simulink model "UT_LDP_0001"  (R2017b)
settings: Solver=FixedStepDiscrete  StartTime=0.0  StopTime=1  FixedStep=0.01  RelTol=1e-3  EnableMultiTasking=on
undefined symbols (not defined in the file): sigbuilder_block
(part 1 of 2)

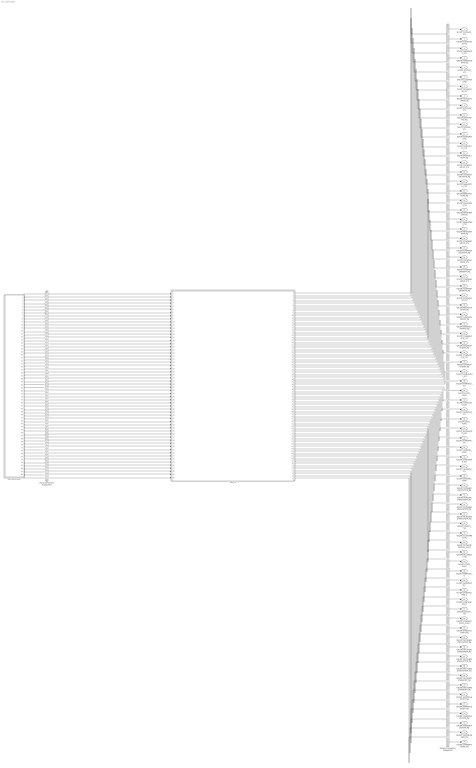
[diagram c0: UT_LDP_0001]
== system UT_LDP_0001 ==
  Harness Inputs : Subsystem  Tag=STV Subsys  LoadFcn=sigbuilder_block('load');  StartFcn=sigbuilder_block('start');  StopFcn=sigbuilder_block('stop');  ClipboardFcn=sigbuilder_block('clipboard');  mask(Sigbuilder block){tuvar=[0:10]}
      mask init:
      | if ~strcmp(get_param(bdroot(gcb),'SimulationStatus'),'stopped'),tuvar = sigbuilder_block('maskInit'); end
  Input Conversion Subsystem : Subsystem  Tag=__SLT_ICS__  Description=Signal spec. and routing
  LDP_UT : ModelReference  ModelNameDialog=LDP_UT  SimulationMode=Normal  ModelReferenceVersion='M104C110'
  Output Conversion Subsystem : Subsystem  Tag=__SLT_OCS__  Description=Signal spec. and routing
  GcLDP_CrntSens_mV : Outport  OutDataTypeStr=uint16  PortDimensions=[1]
  GbLDP_CrntSensVld_flg : Outport  Port=2  OutDataTypeStr=boolean  PortDimensions=[1]
  GcLDP_HallSplyVolt_mV : Outport  Port=3  OutDataTypeStr=uint16  PortDimensions=[1]
  GbLDP_HallSplyVoltVld_flg : Outport  Port=4  OutDataTypeStr=boolean  PortDimensions=[1]
  GcLDP_CC2Volt_mV : Outport  Port=5  OutDataTypeStr=uint16  PortDimensions=[1]
  GbLDP_CC2VoltVld_flg : Outport  Port=6  OutDataTypeStr=boolean  PortDimensions=[1]
  GcLDP_DCSuplyVolt_mV : Outport  Port=7  OutDataTypeStr=uint16  PortDimensions=[1]
  GbLDP_DCSuplyVoltVld_flg : Outport  Port=8  OutDataTypeStr=boolean  PortDimensions=[1]
  GcLDP_Kl30CVolt_mV : Outport  Port=9  OutDataTypeStr=uint16  PortDimensions=[1]
  GbLDP_Kl30CVoltVld_flg : Outport  Port=10  OutDataTypeStr=boolean  PortDimensions=[1]
  GcLDP_Kl30Volt_mV : Outport  Port=11  OutDataTypeStr=uint16  PortDimensions=[1]
  GbLDP_Kl30VoltVld_flg : Outport  Port=12  OutDataTypeStr=boolean  PortDimensions=[1]
  GcLDP_PosHsdCrnt_mV : Outport  Port=13  OutDataTypeStr=uint16  PortDimensions=[1]
  GbLDP_PosHsdCrntVld_flg : Outport  Port=14  OutDataTypeStr=boolean  PortDimensions=[1]
  GcLDP_ChrgPosHsdCrnt_mV : Outport  Port=15  OutDataTypeStr=uint16  PortDimensions=[1]
  GbLDP_ChrgPosHsdCrntVld_flg : Outport  Port=16  OutDataTypeStr=boolean  PortDimensions=[1]
  GcLDP_NegHsdCrnt_mV : Outport  Port=17  OutDataTypeStr=uint16  PortDimensions=[1]
  GbLDP_NegHsdCrntVld_flg : Outport  Port=18  OutDataTypeStr=boolean  PortDimensions=[1]
  GcLDP_PosHsdVolt_mV : Outport  Port=19  OutDataTypeStr=uint16  PortDimensions=[1]
  GbLDP_PosHsdVoltVld_flg : Outport  Port=20  OutDataTypeStr=boolean  PortDimensions=[1]
  GcLDP_NegHsdVolt_mV : Outport  Port=21  OutDataTypeStr=uint16  PortDimensions=[1]
  GbLDP_NegHsdVoltVld_flg : Outport  Port=22  OutDataTypeStr=boolean  PortDimensions=[1]
  GcLDP_ChrgNegHsdCrnt_mV : Outport  Port=23  OutDataTypeStr=uint16  PortDimensions=[1]
  GbLDP_ChrgNegHsdCrntVld_flg : Outport  Port=24  OutDataTypeStr=boolean  PortDimensions=[1]
  GcLDP_ChrgPosHsdVolt_mV : Outport  Port=25  OutDataTypeStr=uint16  PortDimensions=[1]
  GbLDP_ChrgPosHsdVoltVld_flg : Outport  Port=26  OutDataTypeStr=boolean  PortDimensions=[1]
  GcLDP_ChrgNegHsdVolt_mV : Outport  Port=27  OutDataTypeStr=uint16  PortDimensions=[1]
  GbLDP_ChrgNegHsdVoltVld_flg : Outport  Port=28  OutDataTypeStr=boolean  PortDimensions=[1]
  GcLDP_BmuSplyVolt_mV : Outport  Port=29  OutDataTypeStr=uint16  PortDimensions=[1]
  GbLDP_BmuSplyVoltVld_flg : Outport  Port=30  OutDataTypeStr=boolean  PortDimensions=[1]
  GbLDP_lntWtSensVoltVld_flg : Outport  Port=31  OutDataTypeStr=boolean  PortDimensions=[1]
  GbLDP_OutWtSensVoltVld_flg : Outport  Port=32  OutDataTypeStr=boolean  PortDimensions=[1]
  GcLDP_ChrgNegTemp_mV : Outport  Port=33  OutDataTypeStr=uint16  PortDimensions=[1]
  GbLDP_ChrgNegTempVld_flg : Outport  Port=34  OutDataTypeStr=boolean  PortDimensions=[1]
  GcLDP_ChrgPosTemp_mV : Outport  Port=35  OutDataTypeStr=uint16  PortDimensions=[1]
  GbLDP_ChrgPosTempVld_flg : Outport  Port=36  OutDataTypeStr=boolean  PortDimensions=[1]
  GcLDP_HvilDutyOut_pct : Outport  Port=37  OutDataTypeStr=uint8  PortDimensions=[1]
  GcLDP_HvilPerOut_ms : Outport  Port=38  OutDataTypeStr=uint32  PortDimensions=[1]
  GcLDP_HvilSt_numb : Outport  Port=39  OutDataTypeStr=uint8  PortDimensions=[1]
  GcLDP_CshDutyOut_pct : Outport  Port=40  OutDataTypeStr=uint8  PortDimensions=[1]
  GcLDP_CshPerOut_ms : Outport  Port=41  OutDataTypeStr=uint32  PortDimensions=[1]
  GcLDP_CshSt_numb : Outport  Port=42  OutDataTypeStr=uint8  PortDimensions=[1]
  GcLDP_HvilDutyFbkt_pct : Outport  Port=43  OutDataTypeStr=uint8  PortDimensions=[1]
  GcLDP_HvilPerFbk_ms : Outport  Port=44  OutDataTypeStr=uint32  PortDimensions=[1]
  GcLDP_HvilStFbk_numb : Outport  Port=45  OutDataTypeStr=uint8  PortDimensions=[1]
  GcLDP_CshDutyFbk_pct : Outport  Port=46  OutDataTypeStr=uint8  PortDimensions=[1]
  GcLDP_CshPerFbk_ms : Outport  Port=47  OutDataTypeStr=uint32  PortDimensions=[1]
  GcLDP_CshStFbk_numb : Outport  Port=48  OutDataTypeStr=uint8  PortDimensions=[1]
  GbLDP_DCPlugPosTempSTVFlt_flg : Outport  Port=49  OutDataTypeStr=boolean  PortDimensions=[1]
  GbLDP_DCPlugPosTempSTGFlt_flg : Outport  Port=50  OutDataTypeStr=boolean  PortDimensions=[1]
  GbLDP_DCPlugNegTempSTVFlt_flg : Outport  Port=51  OutDataTypeStr=boolean  PortDimensions=[1]
  GbLDP_DCPlugNegTempSTGFlt_flg : Outport  Port=52  OutDataTypeStr=boolean  PortDimensions=[1]
  GbLDP_CC2STG_flg : Outport  Port=53  OutDataTypeStr=boolean  PortDimensions=[1]
  GbLDP_CC2VoltRaty_flg : Outport  Port=54  OutDataTypeStr=boolean  PortDimensions=[1]
  GeLDP_DCPlugTempState_enum : Outport  Port=55  OutDataTypeStr=uint8  PortDimensions=[1]
  GbLDP_DC12VSply_flg : Outport  Port=56  OutDataTypeStr=boolean  PortDimensions=[1]
  GeLDP_CC2St_enum : Outport  Port=57  OutDataTypeStr=uint8  PortDimensions=[1]
  GcLDP_lntWtTemp_C : Outport  Port=58  OutDataTypeStr=single  PortDimensions=[1]
  GcLDP_OutWtTemp_C : Outport  Port=59  OutDataTypeStr=single  PortDimensions=[1]
  GcLDP_ChrgTempNeg_C : Outport  Port=60  OutDataTypeStr=single  PortDimensions=[1]
  GcLDP_ChrgTempPos_C : Outport  Port=61  OutDataTypeStr=single  PortDimensions=[1]
  GbLDP_CC2STV_flg : Outport  Port=62  OutDataTypeStr=boolean  PortDimensions=[1]
  GeLDP_ChrgGunConnSt_enum : Outport  Port=63  OutDataTypeStr=uint8  PortDimensions=[1]
  GbLDP_ChrgGunConnFlt_flg : Outport  Port=64  OutDataTypeStr=boolean  PortDimensions=[1]
  GbLDP_DCChrgPosTempSTVFlt_flg : Outport  Port=65  OutDataTypeStr=boolean  PortDimensions=[1]
  GbLDP_DCChrgPosTempSTGFlt_flg : Outport  Port=66  OutDataTypeStr=boolean  PortDimensions=[1]
  GbLDP_DCChrgNegTempSTVFlt_flg : Outport  Port=67  OutDataTypeStr=boolean  PortDimensions=[1]
  GbLDP_DCChrgNegTempSTGFlt_flg : Outport  Port=68  OutDataTypeStr=boolean  PortDimensions=[1]
  GbLDP_DCChrgPosTempHiFlt_flg : Outport  Port=69  OutDataTypeStr=boolean  PortDimensions=[1]
  GbLDP_DCChrgNegTempHiFlt_flg : Outport  Port=70  OutDataTypeStr=boolean  PortDimensions=[1]
  GbLDP_IntWtTempSTVFlt_flg : Outport  Port=71  OutDataTypeStr=boolean  PortDimensions=[1]
  GbLDP_IntWtTempSTGFlt_flg : Outport  Port=72  OutDataTypeStr=boolean  PortDimensions=[1]
  GbLDP_OutWtTempSTVFlt_flg : Outport  Port=73  OutDataTypeStr=boolean  PortDimensions=[1]
  GbLDP_OutWtTempSTGFlt_flg : Outport  Port=74  OutDataTypeStr=boolean  PortDimensions=[1]
  GbLDP_IntWtTempHiFlt_flg : Outport  Port=75  OutDataTypeStr=boolean  PortDimensions=[1]
  GbLDP_OutWtTempHiFlt_flg : Outport  Port=76  OutDataTypeStr=boolean  PortDimensions=[1]
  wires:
  Harness Inputs/1(GcISP_CrntSens_mV) -> Input Conversion Subsystem/1(Inport_1)
  Harness Inputs/2(GbISP_CrntSensL1Invld_flg) -> Input Conversion Subsystem/2(Inport_2)
  Harness Inputs/3(GbISP_HallSplyVoltVld_flg) -> Input Conversion Subsystem/3(Inport_3)
  Harness Inputs/4(GcISP_HallSplyVolt_mV) -> Input Conversion Subsystem/4(Inport_4)
  Harness Inputs/5(GcISP_CC2Volt_mV) -> Input Conversion Subsystem/5(Inport_5)
  Harness Inputs/6(GbISP_CC2VoltVld_flg) -> Input Conversion Subsystem/6(Inport_6)
  Harness Inputs/7(GcISP_DCSuplyVolt_mV) -> Input Conversion Subsystem/7(Inport_7)
  Harness Inputs/8(GbISP_DCSuplyVoltVld_flg) -> Input Conversion Subsystem/8(Inport_8)
  Harness Inputs/9(GcISP_Kl30CVolt_mV) -> Input Conversion Subsystem/9(Inport_9)
  Harness Inputs/10(GbISP_Kl30CVoltVld_flg) -> Input Conversion Subsystem/10(Inport_10)
  Harness Inputs/11(GbISP_Kl30VoltVld_flg) -> Input Conversion Subsystem/11(Inport_11)
  Harness Inputs/12(GcISP_Kl30Volt_mV) -> Input Conversion Subsystem/12(Inport_12)
  Harness Inputs/13(GcISP_PosHsdCrnt_mV) -> Input Conversion Subsystem/13(Inport_13)
  Harness Inputs/14(GbISP_PosHsdCrntVld_flg) -> Input Conversion Subsystem/14(Inport_14)
  Harness Inputs/15(GcISP_ChrgPosHsdCrnt_mV) -> Input Conversion Subsystem/15(Inport_15)
  Harness Inputs/16(GbISP_ChrgPosHsdCrntVld_flg) -> Input Conversion Subsystem/16(Inport_16)
  Harness Inputs/17(GcISP_NegHsdCrnt_mV) -> Input Conversion Subsystem/17(Inport_17)
  Harness Inputs/18(GbISP_NegHsdCrntVld_flg) -> Input Conversion Subsystem/18(Inport_18)
  Harness Inputs/19(GcISP_PosHsdVolt_mV) -> Input Conversion Subsystem/19(Inport_19)
  Harness Inputs/20(GbISP_PosHsdVoltVld_flg) -> Input Conversion Subsystem/20(Inport_20)
  Harness Inputs/21(GcISP_NegHsdVolt_mV) -> Input Conversion Subsystem/21(Inport_21)
  Harness Inputs/22(GbISP_NegHsdVoltVld_flg) -> Input Conversion Subsystem/22(Inport_22)
  Harness Inputs/23(GcISP_ChrgNegHsdCrnt_mV) -> Input Conversion Subsystem/23(Inport_23)
  Harness Inputs/24(GbISP_ChrgNegHsdCrntVld_flg) -> Input Conversion Subsystem/24(Inport_24)
  Harness Inputs/25(GcISP_ChrgPosHsdVolt_mV) -> Input Conversion Subsystem/25(Inport_25)
  Harness Inputs/26(GbISP_ChrgPosHsdVoltVld_flg) -> Input Conversion Subsystem/26(Inport_26)
  Harness Inputs/27(GcISP_ChrgNegHsdVolt_mV) -> Input Conversion Subsystem/27(Inport_27)
  Harness Inputs/28(GbISP_ChrgNegHsdVoltVld_flg) -> Input Conversion Subsystem/28(Inport_28)
  Harness Inputs/29(GcISP_BmuSplyVolt_mV) -> Input Conversion Subsystem/29(Inport_29)
  Harness Inputs/30(GbISP_BmuSplyVoltVld_flg) -> Input Conversion Subsystem/30(Inport_30)
  Harness Inputs/31(GcISP_lntWtSensVolt_mV) -> Input Conversion Subsystem/31(Inport_31)
  Harness Inputs/32(GbISP_lntWtSensVoltVld_flg) -> Input Conversion Subsystem/32(Inport_32)
  Harness Inputs/33(GcISP_OutWtSensVolt_mV) -> Input Conversion Subsystem/33(Inport_33)
  Harness Inputs/34(GbISP_OutWtSensVoltVld_flg) -> Input Conversion Subsystem/34(Inport_34)
  Harness Inputs/35(GcISP_ChrgNegTemp_mV) -> Input Conversion Subsystem/35(Inport_35)
  Harness Inputs/36(GbISP_ChrgNegTempVld_flg) -> Input Conversion Subsystem/36(Inport_36)
  Harness Inputs/37(GcISP_ChrgPosTemp_mV) -> Input Conversion Subsystem/37(Inport_37)
  Harness Inputs/38(GbISP_ChrgPosTempVld_flg) -> Input Conversion Subsystem/38(Inport_38)
  Harness Inputs/39(GcISP_HvilDutyOut_pct) -> Input Conversion Subsystem/39(Inport_39)
  Harness Inputs/40(GcISP_HvilPerOut_us) -> Input Conversion Subsystem/40(Inport_40)
  Harness Inputs/41(GcISP_HvilSt_numb) -> Input Conversion Subsystem/41(Inport_41)
  Harness Inputs/42(GbISP_HvilOutVld_flg) -> Input Conversion Subsystem/42(Inport_42)
  Harness Inputs/43(GcISP_CshDutyOut_pct) -> Input Conversion Subsystem/43(Inport_43)
  Harness Inputs/44(GcISP_CshPerOut_us) -> Input Conversion Subsystem/44(Inport_44)
  Harness Inputs/45(GcISP_CshSt_numb) -> Input Conversion Subsystem/45(Inport_45)
  Harness Inputs/46(GbISP_CshOutVld_flg) -> Input Conversion Subsystem/46(Inport_46)
  Harness Inputs/47(GcISP_HvilDutyFbkt_pct) -> Input Conversion Subsystem/47(Inport_47)
  Harness Inputs/48(GcISP_HvilPerFbk_us) -> Input Conversion Subsystem/48(Inport_48)
  Harness Inputs/49(GcISP_HvilStFbk_numb) -> Input Conversion Subsystem/49(Inport_49)
  Harness Inputs/50(GbISP_HvilFbkVld_flg) -> Input Conversion Subsystem/50(Inport_50)
  Harness Inputs/51(GcISP_CshDutyFbk_pct) -> Input Conversion Subsystem/51(Inport_51)
  Harness Inputs/52(GcISP_CshPerFbk_us) -> Input Conversion Subsystem/52(Inport_52)
  Harness Inputs/53(GcISP_CshStFbk_numb) -> Input Conversion Subsystem/53(Inport_53)
  Harness Inputs/54(GbISP_CshFbkVld_flg) -> Input Conversion Subsystem/54(Inport_54)
  Harness Inputs/55(GbISP_CrntSensL2Invld_flg) -> Input Conversion Subsystem/55(Inport_55)
  Harness Inputs/56(GeODP_ObcCcSt_enum) -> Input Conversion Subsystem/56(Inport_56)
  Harness Inputs/57(GbISP_TFCC2VoltRaty_flg) -> Input Conversion Subsystem/57(Inport_57)
  Harness Inputs/58(GbISP_TFCC2STV_flg) -> Input Conversion Subsystem/58(Inport_58)
  Harness Inputs/59(GbISP_TFCC2STG_flg) -> Input Conversion Subsystem/59(Inport_59)
  Harness Inputs/60(GeCTC_CtrCtlConnMode_enum) -> Input Conversion Subsystem/60(Inport_60)
  Output Conversion Subsystem/1(Outport_1) -> GcLDP_CrntSens_mV/1
  Output Conversion Subsystem/2(Outport_2) -> GbLDP_CrntSensVld_flg/1
  Output Conversion Subsystem/3(Outport_3) -> GcLDP_HallSplyVolt_mV/1
  Output Conversion Subsystem/4(Outport_4) -> GbLDP_HallSplyVoltVld_flg/1
  Output Conversion Subsystem/5(Outport_5) -> GcLDP_CC2Volt_mV/1
  Output Conversion Subsystem/6(Outport_6) -> GbLDP_CC2VoltVld_flg/1
  Output Conversion Subsystem/7(Outport_7) -> GcLDP_DCSuplyVolt_mV/1
  Output Conversion Subsystem/8(Outport_8) -> GbLDP_DCSuplyVoltVld_flg/1
  Output Conversion Subsystem/9(Outport_9) -> GcLDP_Kl30CVolt_mV/1
  Output Conversion Subsystem/10(Outport_10) -> GbLDP_Kl30CVoltVld_flg/1
  Output Conversion Subsystem/11(Outport_11) -> GcLDP_Kl30Volt_mV/1
  Output Conversion Subsystem/12(Outport_12) -> GbLDP_Kl30VoltVld_flg/1
  Output Conversion Subsystem/13(Outport_13) -> GcLDP_PosHsdCrnt_mV/1
  Output Conversion Subsystem/14(Outport_14) -> GbLDP_PosHsdCrntVld_flg/1
  Output Conversion Subsystem/15(Outport_15) -> GcLDP_ChrgPosHsdCrnt_mV/1
  Output Conversion Subsystem/16(Outport_16) -> GbLDP_ChrgPosHsdCrntVld_flg/1
  Output Conversion Subsystem/17(Outport_17) -> GcLDP_NegHsdCrnt_mV/1
  Output Conversion Subsystem/18(Outport_18) -> GbLDP_NegHsdCrntVld_flg/1
  Output Conversion Subsystem/19(Outport_19) -> GcLDP_PosHsdVolt_mV/1
  Output Conversion Subsystem/20(Outport_20) -> GbLDP_PosHsdVoltVld_flg/1
  Output Conversion Subsystem/21(Outport_21) -> GcLDP_NegHsdVolt_mV/1
  Output Conversion Subsystem/22(Outport_22) -> GbLDP_NegHsdVoltVld_flg/1
  Output Conversion Subsystem/23(Outport_23) -> GcLDP_ChrgNegHsdCrnt_mV/1
  Output Conversion Subsystem/24(Outport_24) -> GbLDP_ChrgNegHsdCrntVld_flg/1
  Output Conversion Subsystem/25(Outport_25) -> GcLDP_ChrgPosHsdVolt_mV/1
  Output Conversion Subsystem/26(Outport_26) -> GbLDP_ChrgPosHsdVoltVld_flg/1
  Output Conversion Subsystem/27(Outport_27) -> GcLDP_ChrgNegHsdVolt_mV/1
  Output Conversion Subsystem/28(Outport_28) -> GbLDP_ChrgNegHsdVoltVld_flg/1
  Output Conversion Subsystem/29(Outport_29) -> GcLDP_BmuSplyVolt_mV/1
  Output Conversion Subsystem/30(Outport_30) -> GbLDP_BmuSplyVoltVld_flg/1
  Output Conversion Subsystem/31(Outport_31) -> GbLDP_lntWtSensVoltVld_flg/1
  Output Conversion Subsystem/32(Outport_32) -> GbLDP_OutWtSensVoltVld_flg/1
  Output Conversion Subsystem/33(Outport_33) -> GcLDP_ChrgNegTemp_mV/1
  Output Conversion Subsystem/34(Outport_34) -> GbLDP_ChrgNegTempVld_flg/1
  Output Conversion Subsystem/35(Outport_35) -> GcLDP_ChrgPosTemp_mV/1
  Output Conversion Subsystem/36(Outport_36) -> GbLDP_ChrgPosTempVld_flg/1
  Output Conversion Subsystem/37(Outport_37) -> GcLDP_HvilDutyOut_pct/1
  Output Conversion Subsystem/38(Outport_38) -> GcLDP_HvilPerOut_ms/1
  Output Conversion Subsystem/39(Outport_39) -> GcLDP_HvilSt_numb/1
  Output Conversion Subsystem/40(Outport_40) -> GcLDP_CshDutyOut_pct/1
  Output Conversion Subsystem/41(Outport_41) -> GcLDP_CshPerOut_ms/1
  Output Conversion Subsystem/42(Outport_42) -> GcLDP_CshSt_numb/1
  Output Conversion Subsystem/43(Outport_43) -> GcLDP_HvilDutyFbkt_pct/1
  Output Conversion Subsystem/44(Outport_44) -> GcLDP_HvilPerFbk_ms/1
  Output Conversion Subsystem/45(Outport_45) -> GcLDP_HvilStFbk_numb/1
  Output Conversion Subsystem/46(Outport_46) -> GcLDP_CshDutyFbk_pct/1
  Output Conversion Subsystem/47(Outport_47) -> GcLDP_CshPerFbk_ms/1
  Output Conversion Subsystem/48(Outport_48) -> GcLDP_CshStFbk_numb/1
  Output Conversion Subsystem/49(Outport_49) -> GbLDP_DCPlugPosTempSTVFlt_flg/1
  Output Conversion Subsystem/50(Outport_50) -> GbLDP_DCPlugPosTempSTGFlt_flg/1
  Output Conversion Subsystem/51(Outport_51) -> GbLDP_DCPlugNegTempSTVFlt_flg/1
  Output Conversion Subsystem/52(Outport_52) -> GbLDP_DCPlugNegTempSTGFlt_flg/1
  Output Conversion Subsystem/53(Outport_53) -> GbLDP_CC2STG_flg/1
  Output Conversion Subsystem/54(Outport_54) -> GbLDP_CC2VoltRaty_flg/1
  Output Conversion Subsystem/55(Outport_55) -> GeLDP_DCPlugTempState_enum/1
  Output Conversion Subsystem/56(Outport_56) -> GbLDP_DC12VSply_flg/1
  Output Conversion Subsystem/57(Outport_57) -> GeLDP_CC2St_enum/1
  Output Conversion Subsystem/58(Outport_58) -> GcLDP_lntWtTemp_C/1
  Output Conversion Subsystem/59(Outport_59) -> GcLDP_OutWtTemp_C/1
  Output Conversion Subsystem/60(Outport_60) -> GcLDP_ChrgTempNeg_C/1
  Output Conversion Subsystem/61(Outport_61) -> GcLDP_ChrgTempPos_C/1
  Output Conversion Subsystem/62(Outport_62) -> GbLDP_CC2STV_flg/1
  Output Conversion Subsystem/63(Outport_63) -> GeLDP_ChrgGunConnSt_enum/1
  Output Conversion Subsystem/64(Outport_64) -> GbLDP_ChrgGunConnFlt_flg/1
  Output Conversion Subsystem/65(Outport_65) -> GbLDP_DCChrgPosTempSTVFlt_flg/1
  Output Conversion Subsystem/66(Outport_66) -> GbLDP_DCChrgPosTempSTGFlt_flg/1
  Output Conversion Subsystem/67(Outport_67) -> GbLDP_DCChrgNegTempSTVFlt_flg/1
  Output Conversion Subsystem/68(Outport_68) -> GbLDP_DCChrgNegTempSTGFlt_flg/1
  Output Conversion Subsystem/69(Outport_69) -> GbLDP_DCChrgPosTempHiFlt_flg/1
  Output Conversion Subsystem/70(Outport_70) -> GbLDP_DCChrgNegTempHiFlt_flg/1
  Output Conversion Subsystem/71(Outport_71) -> GbLDP_IntWtTempSTVFlt_flg/1
  Output Conversion Subsystem/72(Outport_72) -> GbLDP_IntWtTempSTGFlt_flg/1
  Output Conversion Subsystem/73(Outport_73) -> GbLDP_OutWtTempSTVFlt_flg/1
  Output Conversion Subsystem/74(Outport_74) -> GbLDP_OutWtTempSTGFlt_flg/1
  Output Conversion Subsystem/75(Outport_75) -> GbLDP_IntWtTempHiFlt_flg/1
  Output Conversion Subsystem/76(Outport_76) -> GbLDP_OutWtTempHiFlt_flg/1
  Input Conversion Subsystem/1(Outport_1) -> LDP_UT/1
  Input Conversion Subsystem/2(Outport_2) -> LDP_UT/2
  Input Conversion Subsystem/3(Outport_3) -> LDP_UT/3
  Input Conversion Subsystem/4(Outport_4) -> LDP_UT/4
  Input Conversion Subsystem/5(Outport_5) -> LDP_UT/5
  Input Conversion Subsystem/6(Outport_6) -> LDP_UT/6
  Input Conversion Subsystem/7(Outport_7) -> LDP_UT/7
  Input Conversion Subsystem/8(Outport_8) -> LDP_UT/8
  Input Conversion Subsystem/9(Outport_9) -> LDP_UT/9
  Input Conversion Subsystem/10(Outport_10) -> LDP_UT/10
  Input Conversion Subsystem/11(Outport_11) -> LDP_UT/11
  Input Conversion Subsystem/12(Outport_12) -> LDP_UT/12
  Input Conversion Subsystem/13(Outport_13) -> LDP_UT/13
  Input Conversion Subsystem/14(Outport_14) -> LDP_UT/14
  Input Conversion Subsystem/15(Outport_15) -> LDP_UT/15
  Input Conversion Subsystem/16(Outport_16) -> LDP_UT/16
  Input Conversion Subsystem/17(Outport_17) -> LDP_UT/17
  Input Conversion Subsystem/18(Outport_18) -> LDP_UT/18
  Input Conversion Subsystem/19(Outport_19) -> LDP_UT/19
  Input Conversion Subsystem/20(Outport_20) -> LDP_UT/20
  Input Conversion Subsystem/21(Outport_21) -> LDP_UT/21
  Input Conversion Subsystem/22(Outport_22) -> LDP_UT/22
  Input Conversion Subsystem/23(Outport_23) -> LDP_UT/23
  Input Conversion Subsystem/24(Outport_24) -> LDP_UT/24
  Input Conversion Subsystem/25(Outport_25) -> LDP_UT/25
  Input Conversion Subsystem/26(Outport_26) -> LDP_UT/26
  Input Conversion Subsystem/27(Outport_27) -> LDP_UT/27
  Input Conversion Subsystem/28(Outport_28) -> LDP_UT/28
  Input Conversion Subsystem/29(Outport_29) -> LDP_UT/29
  Input Conversion Subsystem/30(Outport_30) -> LDP_UT/30
  Input Conversion Subsystem/31(Outport_31) -> LDP_UT/31
  Input Conversion Subsystem/32(Outport_32) -> LDP_UT/32
  Input Conversion Subsystem/33(Outport_33) -> LDP_UT/33
  Input Conversion Subsystem/34(Outport_34) -> LDP_UT/34
  Input Conversion Subsystem/35(Outport_35) -> LDP_UT/35
  Input Conversion Subsystem/36(Outport_36) -> LDP_UT/36
  Input Conversion Subsystem/37(Outport_37) -> LDP_UT/37
  Input Conversion Subsystem/38(Outport_38) -> LDP_UT/38
  Input Conversion Subsystem/39(Outport_39) -> LDP_UT/39
  Input Conversion Subsystem/40(Outport_40) -> LDP_UT/40
  Input Conversion Subsystem/41(Outport_41) -> LDP_UT/41
  Input Conversion Subsystem/42(Outport_42) -> LDP_UT/42
  Input Conversion Subsystem/43(Outport_43) -> LDP_UT/43
  Input Conversion Subsystem/44(Outport_44) -> LDP_UT/44
  Input Conversion Subsystem/45(Outport_45) -> LDP_UT/45
  Input Conversion Subsystem/46(Outport_46) -> LDP_UT/46
  Input Conversion Subsystem/47(Outport_47) -> LDP_UT/47
  Input Conversion Subsystem/48(Outport_48) -> LDP_UT/48
  Input Conversion Subsystem/49(Outport_49) -> LDP_UT/49
  Input Conversion Subsystem/50(Outport_50) -> LDP_UT/50
  Input Conversion Subsystem/51(Outport_51) -> LDP_UT/51
  Input Conversion Subsystem/52(Outport_52) -> LDP_UT/52
  Input Conversion Subsystem/53(Outport_53) -> LDP_UT/53
  Input Conversion Subsystem/54(Outport_54) -> LDP_UT/54
  Input Conversion Subsystem/55(Outport_55) -> LDP_UT/55
  Input Conversion Subsystem/56(Outport_56) -> LDP_UT/56
  Input Conversion Subsystem/57(Outport_57) -> LDP_UT/57
  Input Conversion Subsystem/58(Outport_58) -> LDP_UT/58
  Input Conversion Subsystem/59(Outport_59) -> LDP_UT/59
  Input Conversion Subsystem/60(Outport_60) -> LDP_UT/60
  LDP_UT/1 -> Output Conversion Subsystem/1(Inport_1)
  LDP_UT/2 -> Output Conversion Subsystem/2(Inport_2)
  LDP_UT/3 -> Output Conversion Subsystem/3(Inport_3)
  LDP_UT/4 -> Output Conversion Subsystem/4(Inport_4)
  LDP_UT/5 -> Output Conversion Subsystem/5(Inport_5)
  LDP_UT/6 -> Output Conversion Subsystem/6(Inport_6)
  LDP_UT/7 -> Output Conversion Subsystem/7(Inport_7)
  LDP_UT/8 -> Output Conversion Subsystem/8(Inport_8)
  LDP_UT/9 -> Output Conversion Subsystem/9(Inport_9)
  LDP_UT/10 -> Output Conversion Subsystem/10(Inport_10)
  LDP_UT/11 -> Output Conversion Subsystem/11(Inport_11)
  LDP_UT/12 -> Output Conversion Subsystem/12(Inport_12)
  LDP_UT/13 -> Output Conversion Subsystem/13(Inport_13)
  LDP_UT/14 -> Output Conversion Subsystem/14(Inport_14)
  LDP_UT/15 -> Output Conversion Subsystem/15(Inport_15)
  LDP_UT/16 -> Output Conversion Subsystem/16(Inport_16)
  LDP_UT/17 -> Output Conversion Subsystem/17(Inport_17)
  LDP_UT/18 -> Output Conversion Subsystem/18(Inport_18)
  LDP_UT/19 -> Output Conversion Subsystem/19(Inport_19)
  LDP_UT/20 -> Output Conversion Subsystem/20(Inport_20)
  LDP_UT/21 -> Output Conversion Subsystem/21(Inport_21)
  LDP_UT/22 -> Output Conversion Subsystem/22(Inport_22)
  LDP_UT/23 -> Output Conversion Subsystem/23(Inport_23)
  LDP_UT/24 -> Output Conversion Subsystem/24(Inport_24)
  LDP_UT/25 -> Output Conversion Subsystem/25(Inport_25)
  LDP_UT/26 -> Output Conversion Subsystem/26(Inport_26)
  LDP_UT/27 -> Output Conversion Subsystem/27(Inport_27)
  LDP_UT/28 -> Output Conversion Subsystem/28(Inport_28)
  LDP_UT/29 -> Output Conversion Subsystem/29(Inport_29)
  LDP_UT/30 -> Output Conversion Subsystem/30(Inport_30)
  LDP_UT/31 -> Output Conversion Subsystem/31(Inport_31)
  LDP_UT/32 -> Output Conversion Subsystem/32(Inport_32)
  LDP_UT/33 -> Output Conversion Subsystem/33(Inport_33)
  LDP_UT/34 -> Output Conversion Subsystem/34(Inport_34)
  LDP_UT/35 -> Output Conversion Subsystem/35(Inport_35)
  LDP_UT/36 -> Output Conversion Subsystem/36(Inport_36)
  LDP_UT/37 -> Output Conversion Subsystem/37(Inport_37)
  LDP_UT/38 -> Output Conversion Subsystem/38(Inport_38)
  LDP_UT/39 -> Output Conversion Subsystem/39(Inport_39)
  LDP_UT/40 -> Output Conversion Subsystem/40(Inport_40)
  LDP_UT/41 -> Output Conversion Subsystem/41(Inport_41)
  LDP_UT/42 -> Output Conversion Subsystem/42(Inport_42)
  LDP_UT/43 -> Output Conversion Subsystem/43(Inport_43)
  LDP_UT/44 -> Output Conversion Subsystem/44(Inport_44)
  LDP_UT/45 -> Output Conversion Subsystem/45(Inport_45)
  LDP_UT/46 -> Output Conversion Subsystem/46(Inport_46)
  LDP_UT/47 -> Output Conversion Subsystem/47(Inport_47)
  LDP_UT/48 -> Output Conversion Subsystem/48(Inport_48)
  LDP_UT/49 -> Output Conversion Subsystem/49(Inport_49)
  LDP_UT/50 -> Output Conversion Subsystem/50(Inport_50)
  LDP_UT/51 -> Output Conversion Subsystem/51(Inport_51)
  LDP_UT/52 -> Output Conversion Subsystem/52(Inport_52)
  LDP_UT/53 -> Output Conversion Subsystem/53(Inport_53)
  LDP_UT/54 -> Output Conversion Subsystem/54(Inport_54)
  LDP_UT/55 -> Output Conversion Subsystem/55(Inport_55)
  LDP_UT/56 -> Output Conversion Subsystem/56(Inport_56)
  LDP_UT/57 -> Output Conversion Subsystem/57(Inport_57)
  LDP_UT/58 -> Output Conversion Subsystem/58(Inport_58)
  LDP_UT/59 -> Output Conversion Subsystem/59(Inport_59)
  LDP_UT/60 -> Output Conversion Subsystem/60(Inport_60)
  LDP_UT/61 -> Output Conversion Subsystem/61(Inport_61)
  LDP_UT/62 -> Output Conversion Subsystem/62(Inport_62)
  LDP_UT/63 -> Output Conversion Subsystem/63(Inport_63)
  LDP_UT/64 -> Output Conversion Subsystem/64(Inport_64)
  LDP_UT/65 -> Output Conversion Subsystem/65(Inport_65)
  LDP_UT/66 -> Output Conversion Subsystem/66(Inport_66)
  LDP_UT/67 -> Output Conversion Subsystem/67(Inport_67)
  LDP_UT/68 -> Output Conversion Subsystem/68(Inport_68)
  LDP_UT/69 -> Output Conversion Subsystem/69(Inport_69)
  LDP_UT/70 -> Output Conversion Subsystem/70(Inport_70)
  LDP_UT/71 -> Output Conversion Subsystem/71(Inport_71)
  LDP_UT/72 -> Output Conversion Subsystem/72(Inport_72)
  LDP_UT/73 -> Output Conversion Subsystem/73(Inport_73)
  LDP_UT/74 -> Output Conversion Subsystem/74(Inport_74)
  LDP_UT/75 -> Output Conversion Subsystem/75(Inport_75)
  LDP_UT/76 -> Output Conversion Subsystem/76(Inport_76)

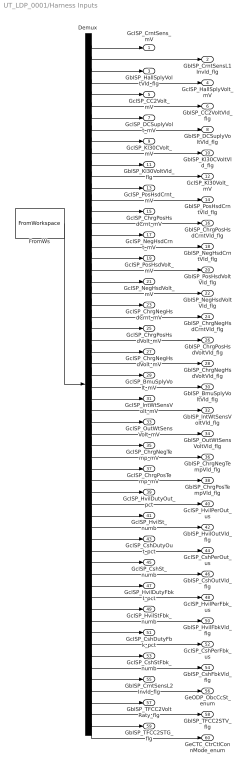
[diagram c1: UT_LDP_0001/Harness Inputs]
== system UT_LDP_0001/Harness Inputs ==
  Demux : Demux  Tag=STV Demux  Outputs=60
  FromWs : FromWorkspace  Tag=STV FromWs  VariableName=tuvar  SampleTime=0
  GcISP_CrntSens_mV : Outport  Tag=STV Outport
  GbISP_CrntSensL1Invld_flg : Outport  Tag=STV Outport  Port=2
  GbISP_HallSplyVoltVld_flg : Outport  Tag=STV Outport  Port=3
  GcISP_HallSplyVolt_mV : Outport  Tag=STV Outport  Port=4
  GcISP_CC2Volt_mV : Outport  Tag=STV Outport  Port=5
  GbISP_CC2VoltVld_flg : Outport  Tag=STV Outport  Port=6
  GcISP_DCSuplyVolt_mV : Outport  Tag=STV Outport  Port=7
  GbISP_DCSuplyVoltVld_flg : Outport  Tag=STV Outport  Port=8
  GcISP_Kl30CVolt_mV : Outport  Tag=STV Outport  Port=9
  GbISP_Kl30CVoltVld_flg : Outport  Tag=STV Outport  Port=10
  GbISP_Kl30VoltVld_flg : Outport  Tag=STV Outport  Port=11
  GcISP_Kl30Volt_mV : Outport  Tag=STV Outport  Port=12
  GcISP_PosHsdCrnt_mV : Outport  Tag=STV Outport  Port=13
  GbISP_PosHsdCrntVld_flg : Outport  Tag=STV Outport  Port=14
  GcISP_ChrgPosHsdCrnt_mV : Outport  Tag=STV Outport  Port=15
  GbISP_ChrgPosHsdCrntVld_flg : Outport  Tag=STV Outport  Port=16
  GcISP_NegHsdCrnt_mV : Outport  Tag=STV Outport  Port=17
  GbISP_NegHsdCrntVld_flg : Outport  Tag=STV Outport  Port=18
  GcISP_PosHsdVolt_mV : Outport  Tag=STV Outport  Port=19
  GbISP_PosHsdVoltVld_flg : Outport  Tag=STV Outport  Port=20
  GcISP_NegHsdVolt_mV : Outport  Tag=STV Outport  Port=21
  GbISP_NegHsdVoltVld_flg : Outport  Tag=STV Outport  Port=22
  GcISP_ChrgNegHsdCrnt_mV : Outport  Tag=STV Outport  Port=23
  GbISP_ChrgNegHsdCrntVld_flg : Outport  Tag=STV Outport  Port=24
  GcISP_ChrgPosHsdVolt_mV : Outport  Tag=STV Outport  Port=25
  GbISP_ChrgPosHsdVoltVld_flg : Outport  Tag=STV Outport  Port=26
  GcISP_ChrgNegHsdVolt_mV : Outport  Tag=STV Outport  Port=27
  GbISP_ChrgNegHsdVoltVld_flg : Outport  Tag=STV Outport  Port=28
  GcISP_BmuSplyVolt_mV : Outport  Tag=STV Outport  Port=29
  GbISP_BmuSplyVoltVld_flg : Outport  Tag=STV Outport  Port=30
  GcISP_lntWtSensVolt_mV : Outport  Tag=STV Outport  Port=31
  GbISP_lntWtSensVoltVld_flg : Outport  Tag=STV Outport  Port=32
  GcISP_OutWtSensVolt_mV : Outport  Tag=STV Outport  Port=33
  GbISP_OutWtSensVoltVld_flg : Outport  Tag=STV Outport  Port=34
  GcISP_ChrgNegTemp_mV : Outport  Tag=STV Outport  Port=35
  GbISP_ChrgNegTempVld_flg : Outport  Tag=STV Outport  Port=36
  GcISP_ChrgPosTemp_mV : Outport  Tag=STV Outport  Port=37
  GbISP_ChrgPosTempVld_flg : Outport  Tag=STV Outport  Port=38
  GcISP_HvilDutyOut_pct : Outport  Tag=STV Outport  Port=39
  GcISP_HvilPerOut_us : Outport  Tag=STV Outport  Port=40
  GcISP_HvilSt_numb : Outport  Tag=STV Outport  Port=41
  GbISP_HvilOutVld_flg : Outport  Tag=STV Outport  Port=42
  GcISP_CshDutyOut_pct : Outport  Tag=STV Outport  Port=43
  GcISP_CshPerOut_us : Outport  Tag=STV Outport  Port=44
  GcISP_CshSt_numb : Outport  Tag=STV Outport  Port=45
  GbISP_CshOutVld_flg : Outport  Tag=STV Outport  Port=46
  GcISP_HvilDutyFbkt_pct : Outport  Tag=STV Outport  Port=47
  GcISP_HvilPerFbk_us : Outport  Tag=STV Outport  Port=48
  GcISP_HvilStFbk_numb : Outport  Tag=STV Outport  Port=49
  GbISP_HvilFbkVld_flg : Outport  Tag=STV Outport  Port=50
  GcISP_CshDutyFbk_pct : Outport  Tag=STV Outport  Port=51
  GcISP_CshPerFbk_us : Outport  Tag=STV Outport  Port=52
  GcISP_CshStFbk_numb : Outport  Tag=STV Outport  Port=53
  GbISP_CshFbkVld_flg : Outport  Tag=STV Outport  Port=54
  GbISP_CrntSensL2Invld_flg : Outport  Tag=STV Outport  Port=55
  GeODP_ObcCcSt_enum : Outport  Tag=STV Outport  Port=56
  GbISP_TFCC2VoltRaty_flg : Outport  Tag=STV Outport  Port=57
  GbISP_TFCC2STV_flg : Outport  Tag=STV Outport  Port=58
  GbISP_TFCC2STG_flg : Outport  Tag=STV Outport  Port=59
  GeCTC_CtrCtlConnMode_enum : Outport  Tag=STV Outport  Port=60
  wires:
  FromWs/1 -> Demux/1
  Demux/1 -> GcISP_CrntSens_mV/1
  Demux/2 -> GbISP_CrntSensL1Invld_flg/1
  Demux/3 -> GbISP_HallSplyVoltVld_flg/1
  Demux/4 -> GcISP_HallSplyVolt_mV/1
  Demux/5 -> GcISP_CC2Volt_mV/1
  Demux/6 -> GbISP_CC2VoltVld_flg/1
  Demux/7 -> GcISP_DCSuplyVolt_mV/1
  Demux/8 -> GbISP_DCSuplyVoltVld_flg/1
  Demux/9 -> GcISP_Kl30CVolt_mV/1
  Demux/10 -> GbISP_Kl30CVoltVld_flg/1
  Demux/11 -> GbISP_Kl30VoltVld_flg/1
  Demux/12 -> GcISP_Kl30Volt_mV/1
  Demux/13 -> GcISP_PosHsdCrnt_mV/1
  Demux/14 -> GbISP_PosHsdCrntVld_flg/1
  Demux/15 -> GcISP_ChrgPosHsdCrnt_mV/1
  Demux/16 -> GbISP_ChrgPosHsdCrntVld_flg/1
  Demux/17 -> GcISP_NegHsdCrnt_mV/1
  Demux/18 -> GbISP_NegHsdCrntVld_flg/1
  Demux/19 -> GcISP_PosHsdVolt_mV/1
  Demux/20 -> GbISP_PosHsdVoltVld_flg/1
  Demux/21 -> GcISP_NegHsdVolt_mV/1
  Demux/22 -> GbISP_NegHsdVoltVld_flg/1
  Demux/23 -> GcISP_ChrgNegHsdCrnt_mV/1
  Demux/24 -> GbISP_ChrgNegHsdCrntVld_flg/1
  Demux/25 -> GcISP_ChrgPosHsdVolt_mV/1
  Demux/26 -> GbISP_ChrgPosHsdVoltVld_flg/1
  Demux/27 -> GcISP_ChrgNegHsdVolt_mV/1
  Demux/28 -> GbISP_ChrgNegHsdVoltVld_flg/1
  Demux/29 -> GcISP_BmuSplyVolt_mV/1
  Demux/30 -> GbISP_BmuSplyVoltVld_flg/1
  Demux/31 -> GcISP_lntWtSensVolt_mV/1
  Demux/32 -> GbISP_lntWtSensVoltVld_flg/1
  Demux/33 -> GcISP_OutWtSensVolt_mV/1
  Demux/34 -> GbISP_OutWtSensVoltVld_flg/1
  Demux/35 -> GcISP_ChrgNegTemp_mV/1
  Demux/36 -> GbISP_ChrgNegTempVld_flg/1
  Demux/37 -> GcISP_ChrgPosTemp_mV/1
  Demux/38 -> GbISP_ChrgPosTempVld_flg/1
  Demux/39 -> GcISP_HvilDutyOut_pct/1
  Demux/40 -> GcISP_HvilPerOut_us/1
  Demux/41 -> GcISP_HvilSt_numb/1
  Demux/42 -> GbISP_HvilOutVld_flg/1
  Demux/43 -> GcISP_CshDutyOut_pct/1
  Demux/44 -> GcISP_CshPerOut_us/1
  Demux/45 -> GcISP_CshSt_numb/1
  Demux/46 -> GbISP_CshOutVld_flg/1
  Demux/47 -> GcISP_HvilDutyFbkt_pct/1
  Demux/48 -> GcISP_HvilPerFbk_us/1
  Demux/49 -> GcISP_HvilStFbk_numb/1
  Demux/50 -> GbISP_HvilFbkVld_flg/1
  Demux/51 -> GcISP_CshDutyFbk_pct/1
  Demux/52 -> GcISP_CshPerFbk_us/1
  Demux/53 -> GcISP_CshStFbk_numb/1
  Demux/54 -> GbISP_CshFbkVld_flg/1
  Demux/55 -> GbISP_CrntSensL2Invld_flg/1
  Demux/56 -> GeODP_ObcCcSt_enum/1
  Demux/57 -> GbISP_TFCC2VoltRaty_flg/1
  Demux/58 -> GbISP_TFCC2STV_flg/1
  Demux/59 -> GbISP_TFCC2STG_flg/1
  Demux/60 -> GeCTC_CtrCtlConnMode_enum/1

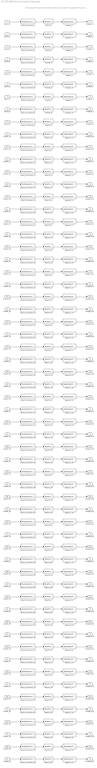
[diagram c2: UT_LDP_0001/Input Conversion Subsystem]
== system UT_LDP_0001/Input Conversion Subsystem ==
  note: This subsystem has been inserted by Simulink to adapt the output of the source blocks to the interface required by the harnessed component. Modifying the contents of this subsystem may result in compilation and simulation failure.
  Inport_1 : Inport
  Inport_2 : Inport  Port=2
  Inport_3 : Inport  Port=3
  Inport_4 : Inport  Port=4
  Inport_5 : Inport  Port=5
  Inport_6 : Inport  Port=6
  Inport_7 : Inport  Port=7
  Inport_8 : Inport  Port=8
  Inport_9 : Inport  Port=9
  Inport_10 : Inport  Port=10
  Inport_11 : Inport  Port=11
  Inport_12 : Inport  Port=12
  Inport_13 : Inport  Port=13
  Inport_14 : Inport  Port=14
  Inport_15 : Inport  Port=15
  Inport_16 : Inport  Port=16
  Inport_17 : Inport  Port=17
  Inport_18 : Inport  Port=18
  Inport_19 : Inport  Port=19
  Inport_20 : Inport  Port=20
  Inport_21 : Inport  Port=21
  Inport_22 : Inport  Port=22
  Inport_23 : Inport  Port=23
  Inport_24 : Inport  Port=24
  Inport_25 : Inport  Port=25
  Inport_26 : Inport  Port=26
  Inport_27 : Inport  Port=27
  Inport_28 : Inport  Port=28
  Inport_29 : Inport  Port=29
  Inport_30 : Inport  Port=30
  Inport_31 : Inport  Port=31
  Inport_32 : Inport  Port=32
  Inport_33 : Inport  Port=33
  Inport_34 : Inport  Port=34
  Inport_35 : Inport  Port=35
  Inport_36 : Inport  Port=36
  Inport_37 : Inport  Port=37
  Inport_38 : Inport  Port=38
  Inport_39 : Inport  Port=39
  Inport_40 : Inport  Port=40
  Inport_41 : Inport  Port=41
  Inport_42 : Inport  Port=42
  Inport_43 : Inport  Port=43
  Inport_44 : Inport  Port=44
  Inport_45 : Inport  Port=45
  Inport_46 : Inport  Port=46
  Inport_47 : Inport  Port=47
  Inport_48 : Inport  Port=48
  Inport_49 : Inport  Port=49
  Inport_50 : Inport  Port=50
  Inport_51 : Inport  Port=51
  Inport_52 : Inport  Port=52
  Inport_53 : Inport  Port=53
  Inport_54 : Inport  Port=54
  Inport_55 : Inport  Port=55
  Inport_56 : Inport  Port=56
  Inport_57 : Inport  Port=57
  Inport_58 : Inport  Port=58
  Inport_59 : Inport  Port=59
  Inport_60 : Inport  Port=60
  Data_Conversion_{1,4..5,13,15,17,19,21,23,25,27,31,33,35,37} (15 alike) : DataTypeConversion  OutDataTypeStr=fixdt('ufix16_Sp2')
  Data_Conversion_{2..3,6,8,10..11,14,16,18,20,22,24,26,28,30,32,34,36,38,42,46,50,54..55,57..59} (27 alike) : DataTypeConversion  OutDataTypeStr=boolean
  Data_Conversion_{7,9,12,29} (4 alike) : DataTypeConversion  OutDataTypeStr=uint16
  Data_Conversion_{39,43,47,51} (4 alike) : DataTypeConversion  OutDataTypeStr=fixdt('ufix32_Sp0030517578125')
  Data_Conversion_{40,44,48,52} (4 alike) : DataTypeConversion  OutDataTypeStr=fixdt('ufix32_Sp001')
  Data_Conversion_{41,45,49,53,56,60} (6 alike) : DataTypeConversion  OutDataTypeStr=uint8
  RateTs_{1..60} (60 alike) : RateTransition  OutPortSampleTime=0.01
  SigSpec_{1,4..5,13,15,17,19,21,23,25,27,31,33,35,37} (15 alike) : SignalSpecification  OutDataTypeStr=fixdt('ufix16_Sp2')  Unit=mV  Dimensions=[1]  SampleTime=0.01
  SigSpec_{2..3,6,8,10..11,14,16,18,20,22,24,26,28,30,32,34,36,38,42,46,50,54..55,57..59} (27 alike) : SignalSpecification  OutDataTypeStr=boolean  Unit=flag  Dimensions=[1]  SampleTime=0.01
  SigSpec_{7,9,12,29} (4 alike) : SignalSpecification  OutDataTypeStr=uint16  Unit=mV  Dimensions=[1]  SampleTime=0.01
  SigSpec_{39,43,47,51} (4 alike) : SignalSpecification  OutDataTypeStr=fixdt('ufix32_Sp0030517578125')  Unit=%  Dimensions=[1]  SampleTime=0.01
  SigSpec_{40,44,48,52} (4 alike) : SignalSpecification  OutDataTypeStr=fixdt('ufix32_Sp001')  Unit=us  Dimensions=[1]  SampleTime=0.01
  SigSpec_41 : SignalSpecification  OutDataTypeStr=uint8  Unit=NA  Dimensions=[1]  SampleTime=0.01
  SigSpec_45 : SignalSpecification  OutDataTypeStr=uint8  Unit=NA  Dimensions=[1]  SampleTime=0.01
  SigSpec_49 : SignalSpecification  OutDataTypeStr=uint8  Unit=numb  Dimensions=[1]  SampleTime=0.01
  SigSpec_53 : SignalSpecification  OutDataTypeStr=uint8  Unit=numb  Dimensions=[1]  SampleTime=0.01
  SigSpec_56 : SignalSpecification  OutDataTypeStr=uint8  Unit=numb  Dimensions=[1]  SampleTime=0.01
  SigSpec_60 : SignalSpecification  OutDataTypeStr=uint8  Unit=enum  Dimensions=[1]  SampleTime=0.01
  Outport_1 : Outport
  Outport_2 : Outport  Port=2
  Outport_3 : Outport  Port=3
  Outport_4 : Outport  Port=4
  Outport_5 : Outport  Port=5
  Outport_6 : Outport  Port=6
  Outport_7 : Outport  Port=7
  Outport_8 : Outport  Port=8
  Outport_9 : Outport  Port=9
  Outport_10 : Outport  Port=10
  Outport_11 : Outport  Port=11
  Outport_12 : Outport  Port=12
  Outport_13 : Outport  Port=13
  Outport_14 : Outport  Port=14
  Outport_15 : Outport  Port=15
  Outport_16 : Outport  Port=16
  Outport_17 : Outport  Port=17
  Outport_18 : Outport  Port=18
  Outport_19 : Outport  Port=19
  Outport_20 : Outport  Port=20
  Outport_21 : Outport  Port=21
  Outport_22 : Outport  Port=22
  Outport_23 : Outport  Port=23
  Outport_24 : Outport  Port=24
  Outport_25 : Outport  Port=25
  Outport_26 : Outport  Port=26
  Outport_27 : Outport  Port=27
  Outport_28 : Outport  Port=28
  Outport_29 : Outport  Port=29
  Outport_30 : Outport  Port=30
  Outport_31 : Outport  Port=31
  Outport_32 : Outport  Port=32
  Outport_33 : Outport  Port=33
  Outport_34 : Outport  Port=34
  Outport_35 : Outport  Port=35
  Outport_36 : Outport  Port=36
  Outport_37 : Outport  Port=37
  Outport_38 : Outport  Port=38
  Outport_39 : Outport  Port=39
  Outport_40 : Outport  Port=40
  Outport_41 : Outport  Port=41
  Outport_42 : Outport  Port=42
  Outport_43 : Outport  Port=43
  Outport_44 : Outport  Port=44
  Outport_45 : Outport  Port=45
  Outport_46 : Outport  Port=46
  Outport_47 : Outport  Port=47
  Outport_48 : Outport  Port=48
  Outport_49 : Outport  Port=49
  Outport_50 : Outport  Port=50
  Outport_51 : Outport  Port=51
  Outport_52 : Outport  Port=52
  Outport_53 : Outport  Port=53
  Outport_54 : Outport  Port=54
  Outport_55 : Outport  Port=55
  Outport_56 : Outport  Port=56
  Outport_57 : Outport  Port=57
  Outport_58 : Outport  Port=58
  Outport_59 : Outport  Port=59
  Outport_60 : Outport  Port=60
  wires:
  SigSpec_1/1 -> Outport_1/1
  RateTs_1/1 -> SigSpec_1/1
  Data_Conversion_1/1 -> RateTs_1/1
  Inport_1/1 -> Data_Conversion_1/1
  SigSpec_2/1 -> Outport_2/1
  RateTs_2/1 -> SigSpec_2/1
  Data_Conversion_2/1 -> RateTs_2/1
  Inport_2/1 -> Data_Conversion_2/1
  SigSpec_3/1 -> Outport_3/1
  RateTs_3/1 -> SigSpec_3/1
  Data_Conversion_3/1 -> RateTs_3/1
  Inport_3/1 -> Data_Conversion_3/1
  SigSpec_4/1 -> Outport_4/1
  RateTs_4/1 -> SigSpec_4/1
  Data_Conversion_4/1 -> RateTs_4/1
  Inport_4/1 -> Data_Conversion_4/1
  SigSpec_5/1 -> Outport_5/1
  RateTs_5/1 -> SigSpec_5/1
  Data_Conversion_5/1 -> RateTs_5/1
  Inport_5/1 -> Data_Conversion_5/1
  SigSpec_6/1 -> Outport_6/1
  RateTs_6/1 -> SigSpec_6/1
  Data_Conversion_6/1 -> RateTs_6/1
  Inport_6/1 -> Data_Conversion_6/1
  SigSpec_7/1 -> Outport_7/1
  RateTs_7/1 -> SigSpec_7/1
  Data_Conversion_7/1 -> RateTs_7/1
  Inport_7/1 -> Data_Conversion_7/1
  SigSpec_8/1 -> Outport_8/1
  RateTs_8/1 -> SigSpec_8/1
  Data_Conversion_8/1 -> RateTs_8/1
  Inport_8/1 -> Data_Conversion_8/1
  SigSpec_9/1 -> Outport_9/1
  RateTs_9/1 -> SigSpec_9/1
  Data_Conversion_9/1 -> RateTs_9/1
  Inport_9/1 -> Data_Conversion_9/1
  SigSpec_10/1 -> Outport_10/1
  RateTs_10/1 -> SigSpec_10/1
  Data_Conversion_10/1 -> RateTs_10/1
  Inport_10/1 -> Data_Conversion_10/1
  SigSpec_11/1 -> Outport_11/1
  RateTs_11/1 -> SigSpec_11/1
  Data_Conversion_11/1 -> RateTs_11/1
  Inport_11/1 -> Data_Conversion_11/1
  SigSpec_12/1 -> Outport_12/1
  RateTs_12/1 -> SigSpec_12/1
  Data_Conversion_12/1 -> RateTs_12/1
  Inport_12/1 -> Data_Conversion_12/1
  SigSpec_13/1 -> Outport_13/1
  RateTs_13/1 -> SigSpec_13/1
  Data_Conversion_13/1 -> RateTs_13/1
  Inport_13/1 -> Data_Conversion_13/1
  SigSpec_14/1 -> Outport_14/1
  RateTs_14/1 -> SigSpec_14/1
  Data_Conversion_14/1 -> RateTs_14/1
  Inport_14/1 -> Data_Conversion_14/1
  SigSpec_15/1 -> Outport_15/1
  RateTs_15/1 -> SigSpec_15/1
  Data_Conversion_15/1 -> RateTs_15/1
  Inport_15/1 -> Data_Conversion_15/1
  SigSpec_16/1 -> Outport_16/1
  RateTs_16/1 -> SigSpec_16/1
  Data_Conversion_16/1 -> RateTs_16/1
  Inport_16/1 -> Data_Conversion_16/1
  SigSpec_17/1 -> Outport_17/1
  RateTs_17/1 -> SigSpec_17/1
  Data_Conversion_17/1 -> RateTs_17/1
  Inport_17/1 -> Data_Conversion_17/1
  SigSpec_18/1 -> Outport_18/1
  RateTs_18/1 -> SigSpec_18/1
  Data_Conversion_18/1 -> RateTs_18/1
  Inport_18/1 -> Data_Conversion_18/1
  SigSpec_19/1 -> Outport_19/1
  RateTs_19/1 -> SigSpec_19/1
  Data_Conversion_19/1 -> RateTs_19/1
  Inport_19/1 -> Data_Conversion_19/1
  SigSpec_20/1 -> Outport_20/1
  RateTs_20/1 -> SigSpec_20/1
  Data_Conversion_20/1 -> RateTs_20/1
  Inport_20/1 -> Data_Conversion_20/1
  SigSpec_21/1 -> Outport_21/1
  RateTs_21/1 -> SigSpec_21/1
  Data_Conversion_21/1 -> RateTs_21/1
  Inport_21/1 -> Data_Conversion_21/1
  SigSpec_22/1 -> Outport_22/1
  RateTs_22/1 -> SigSpec_22/1
  Data_Conversion_22/1 -> RateTs_22/1
  Inport_22/1 -> Data_Conversion_22/1
  SigSpec_23/1 -> Outport_23/1
  RateTs_23/1 -> SigSpec_23/1
  Data_Conversion_23/1 -> RateTs_23/1
  Inport_23/1 -> Data_Conversion_23/1
  SigSpec_24/1 -> Outport_24/1
  RateTs_24/1 -> SigSpec_24/1
  Data_Conversion_24/1 -> RateTs_24/1
  Inport_24/1 -> Data_Conversion_24/1
  SigSpec_25/1 -> Outport_25/1
  RateTs_25/1 -> SigSpec_25/1
  Data_Conversion_25/1 -> RateTs_25/1
  Inport_25/1 -> Data_Conversion_25/1
  SigSpec_26/1 -> Outport_26/1
  RateTs_26/1 -> SigSpec_26/1
  Data_Conversion_26/1 -> RateTs_26/1
  Inport_26/1 -> Data_Conversion_26/1
  SigSpec_27/1 -> Outport_27/1
  RateTs_27/1 -> SigSpec_27/1
  Data_Conversion_27/1 -> RateTs_27/1
  Inport_27/1 -> Data_Conversion_27/1
  SigSpec_28/1 -> Outport_28/1
  RateTs_28/1 -> SigSpec_28/1
  Data_Conversion_28/1 -> RateTs_28/1
  Inport_28/1 -> Data_Conversion_28/1
  SigSpec_29/1 -> Outport_29/1
  RateTs_29/1 -> SigSpec_29/1
  Data_Conversion_29/1 -> RateTs_29/1
  Inport_29/1 -> Data_Conversion_29/1
  SigSpec_30/1 -> Outport_30/1
  RateTs_30/1 -> SigSpec_30/1
  Data_Conversion_30/1 -> RateTs_30/1
  Inport_30/1 -> Data_Conversion_30/1
  SigSpec_31/1 -> Outport_31/1
  RateTs_31/1 -> SigSpec_31/1
  Data_Conversion_31/1 -> RateTs_31/1
  Inport_31/1 -> Data_Conversion_31/1
  SigSpec_32/1 -> Outport_32/1
  RateTs_32/1 -> SigSpec_32/1
  Data_Conversion_32/1 -> RateTs_32/1
  Inport_32/1 -> Data_Conversion_32/1
  SigSpec_33/1 -> Outport_33/1
  RateTs_33/1 -> SigSpec_33/1
  Data_Conversion_33/1 -> RateTs_33/1
  Inport_33/1 -> Data_Conversion_33/1
  SigSpec_34/1 -> Outport_34/1
  RateTs_34/1 -> SigSpec_34/1
  Data_Conversion_34/1 -> RateTs_34/1
  Inport_34/1 -> Data_Conversion_34/1
  SigSpec_35/1 -> Outport_35/1
  RateTs_35/1 -> SigSpec_35/1
  Data_Conversion_35/1 -> RateTs_35/1
  Inport_35/1 -> Data_Conversion_35/1
  SigSpec_36/1 -> Outport_36/1
  RateTs_36/1 -> SigSpec_36/1
  Data_Conversion_36/1 -> RateTs_36/1
  Inport_36/1 -> Data_Conversion_36/1
  SigSpec_37/1 -> Outport_37/1
  RateTs_37/1 -> SigSpec_37/1
  Data_Conversion_37/1 -> RateTs_37/1
  Inport_37/1 -> Data_Conversion_37/1
  SigSpec_38/1 -> Outport_38/1
  RateTs_38/1 -> SigSpec_38/1
  Data_Conversion_38/1 -> RateTs_38/1
  Inport_38/1 -> Data_Conversion_38/1
  SigSpec_39/1 -> Outport_39/1
  RateTs_39/1 -> SigSpec_39/1
  Data_Conversion_39/1 -> RateTs_39/1
  Inport_39/1 -> Data_Conversion_39/1
  SigSpec_40/1 -> Outport_40/1
  RateTs_40/1 -> SigSpec_40/1
  Data_Conversion_40/1 -> RateTs_40/1
  Inport_40/1 -> Data_Conversion_40/1
  SigSpec_41/1 -> Outport_41/1
  RateTs_41/1 -> SigSpec_41/1
  Data_Conversion_41/1 -> RateTs_41/1
  Inport_41/1 -> Data_Conversion_41/1
  SigSpec_42/1 -> Outport_42/1
  RateTs_42/1 -> SigSpec_42/1
  Data_Conversion_42/1 -> RateTs_42/1
  Inport_42/1 -> Data_Conversion_42/1
  SigSpec_43/1 -> Outport_43/1
  RateTs_43/1 -> SigSpec_43/1
  Data_Conversion_43/1 -> RateTs_43/1
  Inport_43/1 -> Data_Conversion_43/1
  SigSpec_44/1 -> Outport_44/1
  RateTs_44/1 -> SigSpec_44/1
  Data_Conversion_44/1 -> RateTs_44/1
  Inport_44/1 -> Data_Conversion_44/1
  SigSpec_45/1 -> Outport_45/1
  RateTs_45/1 -> SigSpec_45/1
  Data_Conversion_45/1 -> RateTs_45/1
  Inport_45/1 -> Data_Conversion_45/1
  SigSpec_46/1 -> Outport_46/1
  RateTs_46/1 -> SigSpec_46/1
  Data_Conversion_46/1 -> RateTs_46/1
  Inport_46/1 -> Data_Conversion_46/1
  SigSpec_47/1 -> Outport_47/1
  RateTs_47/1 -> SigSpec_47/1
  Data_Conversion_47/1 -> RateTs_47/1
  Inport_47/1 -> Data_Conversion_47/1
  SigSpec_48/1 -> Outport_48/1
  RateTs_48/1 -> SigSpec_48/1
  Data_Conversion_48/1 -> RateTs_48/1
  Inport_48/1 -> Data_Conversion_48/1
  SigSpec_49/1 -> Outport_49/1
  RateTs_49/1 -> SigSpec_49/1
  Data_Conversion_49/1 -> RateTs_49/1
  Inport_49/1 -> Data_Conversion_49/1
  SigSpec_50/1 -> Outport_50/1
  RateTs_50/1 -> SigSpec_50/1
  Data_Conversion_50/1 -> RateTs_50/1
  Inport_50/1 -> Data_Conversion_50/1
  SigSpec_51/1 -> Outport_51/1
  RateTs_51/1 -> SigSpec_51/1
  Data_Conversion_51/1 -> RateTs_51/1
  Inport_51/1 -> Data_Conversion_51/1
  SigSpec_52/1 -> Outport_52/1
  RateTs_52/1 -> SigSpec_52/1
  Data_Conversion_52/1 -> RateTs_52/1
  Inport_52/1 -> Data_Conversion_52/1
  SigSpec_53/1 -> Outport_53/1
  RateTs_53/1 -> SigSpec_53/1
  Data_Conversion_53/1 -> RateTs_53/1
  Inport_53/1 -> Data_Conversion_53/1
  SigSpec_54/1 -> Outport_54/1
  RateTs_54/1 -> SigSpec_54/1
  Data_Conversion_54/1 -> RateTs_54/1
  Inport_54/1 -> Data_Conversion_54/1
  SigSpec_55/1 -> Outport_55/1
  RateTs_55/1 -> SigSpec_55/1
  Data_Conversion_55/1 -> RateTs_55/1
  Inport_55/1 -> Data_Conversion_55/1
  SigSpec_56/1 -> Outport_56/1
  RateTs_56/1 -> SigSpec_56/1
  Data_Conversion_56/1 -> RateTs_56/1
  Inport_56/1 -> Data_Conversion_56/1
  SigSpec_57/1 -> Outport_57/1
  RateTs_57/1 -> SigSpec_57/1
  Data_Conversion_57/1 -> RateTs_57/1
  Inport_57/1 -> Data_Conversion_57/1
  SigSpec_58/1 -> Outport_58/1
  RateTs_58/1 -> SigSpec_58/1
  Data_Conversion_58/1 -> RateTs_58/1
  Inport_58/1 -> Data_Conversion_58/1
  SigSpec_59/1 -> Outport_59/1
  RateTs_59/1 -> SigSpec_59/1
  Data_Conversion_59/1 -> RateTs_59/1
  Inport_59/1 -> Data_Conversion_59/1
  SigSpec_60/1 -> Outport_60/1
  RateTs_60/1 -> SigSpec_60/1
  Data_Conversion_60/1 -> RateTs_60/1
  Inport_60/1 -> Data_Conversion_60/1
